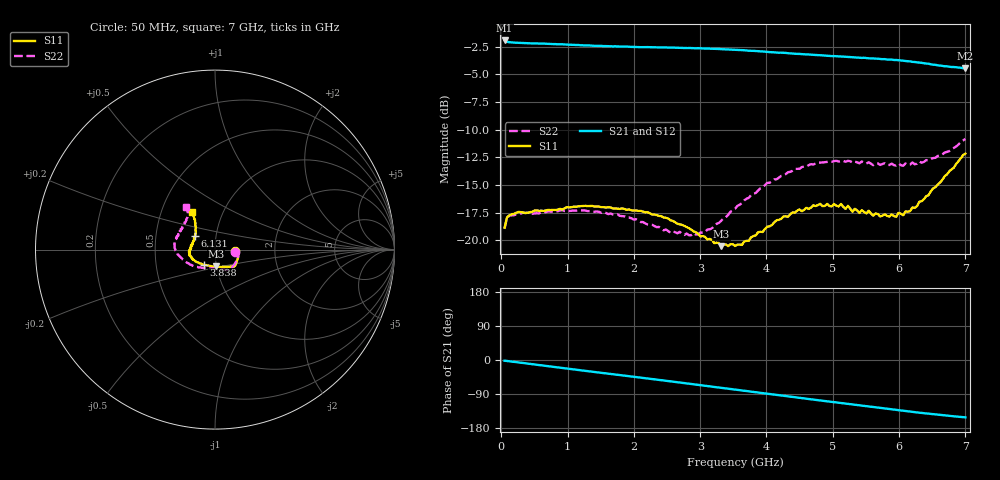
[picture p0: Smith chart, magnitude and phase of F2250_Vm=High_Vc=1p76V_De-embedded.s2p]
! Integrated Device Technology
! Corporate Headquarters
! 6024 Silver Creek Valley Road
! San Jose, CA 95138  USA
! Phone:  1-408-284-8200
! Toll Free:  1-800-223-1366
! Webpage:  http://www.idt.com/
! Timing and RF Division
! 515 Groton Road, Suite 102
! Westford, MA 01886-6024
! Device:  F2250
! Description: Voltage Variable RF Attenuator
! Frequency:  50.0 -  6000.00 MHz
! Package:  3x3 mm Thin QFN Plastic Package: 16 pin
! Ports:  2 RF, 3 DC
!  Pin  1  = GND
!  Pin  2  = NC
!  Pin  3  = RF1  = Port 1
!  Pin  4  = NC
!  Pin  5  = GND
!  Pin  6  = GND
!  Pin  7  = GND
!  Pin  8  = GND
!  Pin  9  = NC
!  Pin 10  = RF2  = Port 2
!  Pin 11  = NC
!  Pin 12  = GND
!  Pin 13  = GND
!  Pin 14  = VCNTRL
!  Pin 15  = VDD
!  Pin 16  = VMODE
! Vcntrl:  1.760 Volts
! Vmode:  +3.300 Volts
! Vdd:  +3.30  Volts
! Current:  1.326 mA
! Data:  The device was measured on a the F2250 evaluation board which has
!  individual transmission lines to the RF pins.  Data was collected
!  using a calibrated network analyzer.  The evaluation board was
!  de-embedded using a TRL calibration technique.
!  The reference plane is the edge of the package pin.
! Misc:  SN 10
!  Action Tracker AT0258
! Date Measured:  2014-11-26
! Date:  2015-10-15  MJV
! Note:
!  Integrated Device Technology supplies this data as a sample of measured
!  data at the package pin for this product.  Your particular data for this
!  product may vary.
!  Data was taken at 25 degrees C.
!  Integrated Device Technology reserves the right to change this data at anytime.
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# GHz S dB R 50
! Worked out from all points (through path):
!   201 points, 50 MHz to 7 GHz, reference 50 ohm
!   highest |S21| = -1.95 dB at 50 MHz (marker M1); lowest = -4.5 dB at 7 GHz (marker M2)
!   group delay of S21, straight-line fit = 60.8 ps
!   lowest |S11| = -20.5 dB at 3.317 GHz (marker M3), VSWR 1.21, Z = 49.6 - j9.41 ohm
!   |S11| at or under -10 dB: start of sweep to end of sweep
!   |S22| runs from -19.5 to -10.8 dB; largest |S21 - S12| = 0.0028
!   S11 on the Smith chart (normalised r, x): 50 MHz: 1.26, -0.02; 3.838 GHz: 0.87, -0.15; 6.131 GHz: 0.79, +0.12; 7 GHz: 0.71, +0.32
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0.05  -18.85 -4.5  -1.95 -1.9  -1.95 -1.9  -18.92 -5.9
0.08475  -17.92 -4.3  -2.07 -2.6  -2.05 -2.5  -17.97 -5.7
0.2585  -17.43 -10.2  -2.16 -6.4  -2.16 -6.4  -17.65 -12.8
1.2315  -16.90 -37.3  -2.39 -27.9  -2.39 -27.9  -17.29 -48.7
1.75275  -17.13 -44.1  -2.49 -39.0  -2.48 -39.0  -17.64 -60.2
2.37825  -17.79 -47.8  -2.58 -52.4  -2.57 -52.5  -18.79 -72.9
2.86475  -19.03 -58.8  -2.63 -63.2  -2.64 -63.2  -19.53 -94.7
3.07325  -19.68 -69.2  -2.68 -67.9  -2.67 -67.9  -19.24 -108.2
3.3165  -20.52 -87.1  -2.74 -73.5  -2.73 -73.5  -18.23 -124.2
3.525  -20.50 -103.8  -2.79 -78.2  -2.80 -78.2  -17.15 -136.0
3.83775  -19.55 -127.3  -2.90 -85.2  -2.90 -85.3  -15.72 -151.0
4.32425  -17.87 -151.7  -3.10 -96.0  -3.11 -96.0  -13.85 -169.7
4.7065  -16.83 -165.2  -3.24 -104.4  -3.23 -104.4  -13.14 -179.7
5.1235  -16.71 -175.9  -3.40 -113.5  -3.39 -113.6  -12.82 170.2
5.29725  -17.42 178.9  -3.46 -117.2  -3.45 -117.3  -12.97 166.8
5.332  -17.15 177.4  -3.48 -118.1  -3.46 -118.1  -12.88 165.8
5.4015  -17.53 175.9  -3.51 -119.6  -3.49 -119.6  -13.04 163.8
5.5405  -17.32 170.1  -3.56 -122.6  -3.53 -122.7  -12.95 160.1
5.85325  -17.84 158.4  -3.68 -129.3  -3.66 -129.4  -13.19 151.9
6.13125  -17.41 145.1  -3.82 -135.3  -3.82 -135.4  -13.17 144.2
6.54825  -15.19 129.5  -4.15 -143.9  -4.14 -144.0  -12.54 130.7
7  -12.17 122.0  -4.46 -151.3  -4.46 -151.4  -10.84 124.0
